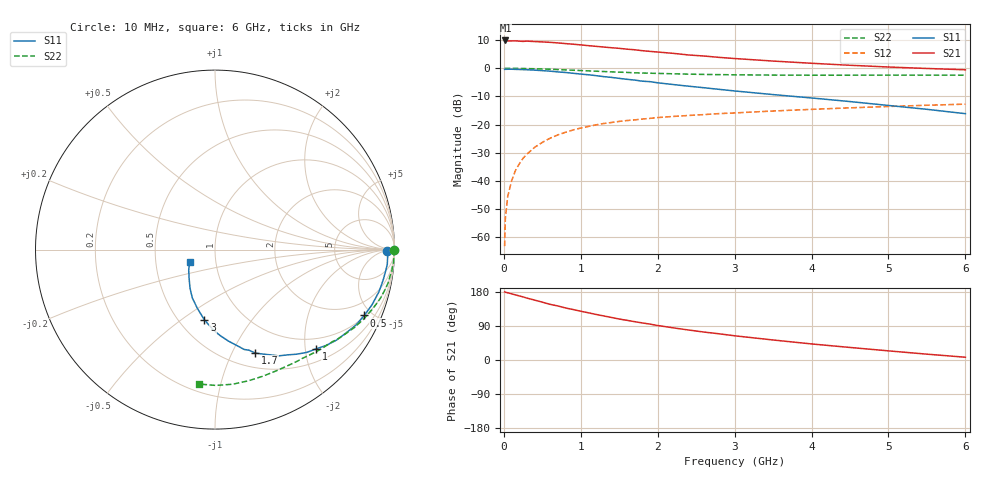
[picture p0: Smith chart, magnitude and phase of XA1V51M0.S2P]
! SIEMENS Discrete & RF Semiconductors
! BFY180
! Si NPN RF Bipolar Junction Transistor in MICRO-X
! VCE = 1.5 V  IC = 1 mA
! Common Emitter S-Parameters:  May  1997
# GHz  S  MA  R  50
!  f  S11  S21  S12  S22
! GHz  MAG  ANG  MAG  ANG  MAG  ANG  MAG  ANG
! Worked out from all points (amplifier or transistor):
!   36 points, 10 MHz to 6 GHz, reference 50 ohm
!   highest |S21| = 9.9 dB at 20 MHz (marker M1)
!   |S21| within 3 dB of that: start of sweep to 1.57 GHz
!   unconditionally stable (mu >= 1): 3.421 GHz to end of sweep
!   at 250 MHz: K = 0.08, MSG = 20.7 dB, |S12| = -31.9 dB
!   at 1.4 GHz: K = 0.54, MSG = 13.3 dB, |S12| = -19.2 dB
!   at 6 GHz: K = 1.08, MAG = 4.3 dB, |S12| = -12.7 dB
!   S11 on the Smith chart (normalised r, x): 10 MHz: 48, -6; 500 MHz: 1.07, -4.50; 1 GHz: 0.76, -2.23; 1.7 GHz: 0.66, -1.24; 3 GHz: 0.66, -0.62; 6 GHz: 0.75, -0.10
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0.01  0.9595 -0.3  3.037 179.7  0.0007 95.2  0.9974 -0.2
0.02  0.9596 -1.0  3.118 178.8  0.0022 96.7  0.9999 -0.5
0.05  0.9627 -2.3  3.058 177.4  0.0053 87.4  0.9978 -1.4
0.1  0.9634 -5.0  3.06 174.7  0.01 86.0  0.9971 -2.8
0.15  0.9574 -7.5  3.073 171.9  0.0153 86.2  0.997 -4.2
0.25  0.948 -12.1  3.001 166.6  0.0254 82.1  0.9926 -7.0
0.3  0.9428 -14.5  3.034 163.3  0.0301 80.0  0.9871 -8.3
0.5  0.909 -23.8  2.937 152.6  0.0485 73.9  0.9719 -13.6
0.6  0.8907 -28.2  2.888 146.9  0.0574 70.7  0.9621 -16.1
0.8  0.8434 -36.8  2.743 137.4  0.0732 64.6  0.937 -20.8
1  0.7898 -44.4  2.601 128.7  0.0872 59.2  0.9131 -25.3
1.1  0.7674 -48.3  2.521 124.5  0.093 57.1  0.9008 -27.2
1.5  0.663 -62.2  2.259 108.1  0.1143 48.9  0.8542 -34.7
1.7  0.6186 -68.7  2.131 101.2  0.1215 45.7  0.8322 -37.9
2  0.5529 -76.6  1.943 91.0  0.1337 41.6  0.8122 -42.6
2.2  0.5155 -81.6  1.843 84.9  0.14 38.9  0.7992 -45.6
2.6  0.4522 -90.6  1.652 73.8  0.151 34.8  0.7783 -50.9
3  0.3965 -98.5  1.49 63.9  0.1615 31.1  0.7664 -56.2
3.5  0.3417 -106.7  1.344 52.8  0.1748 27.2  0.7576 -62.5
4.5  0.2571 -122.7  1.132 33.1  0.199 19.3  0.7544 -75.7
5.5  0.1872 -141.5  0.993 15.4  0.2211 11.5  0.7567 -89.7
6  0.1568 -154.6  0.941 7.3  0.2312 7.2  0.7542 -96.7
